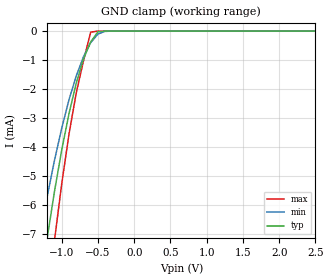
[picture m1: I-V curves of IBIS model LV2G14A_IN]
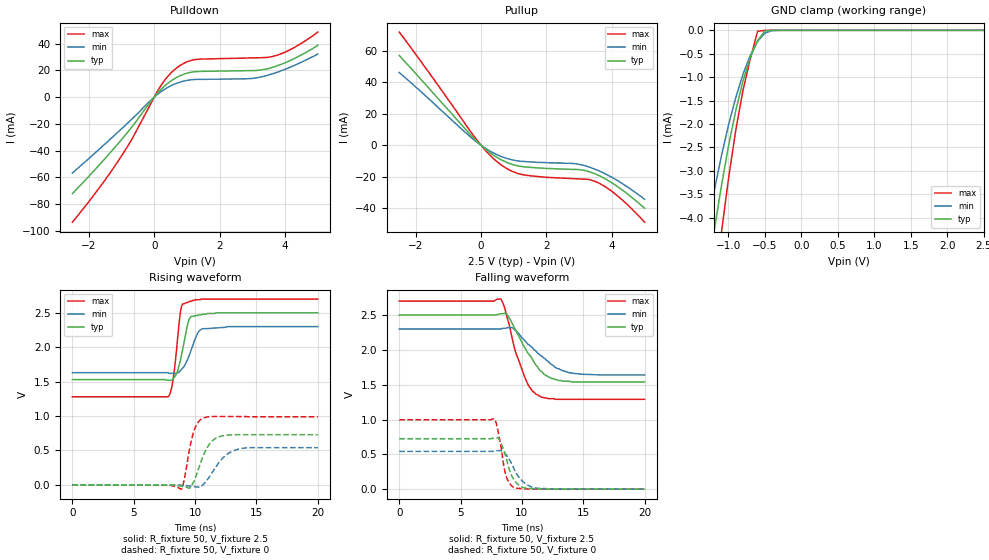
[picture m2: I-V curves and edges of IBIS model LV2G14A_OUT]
|/_/_/_/_/_/_/_/_/_/_/_/_/_/_/_/_/_/_/_/_/_/_/_/_/_/_/_/_/_/_/_/_/_/_/_/_/_/
|   Renesas Electronics Corp.
|   Multi Purpose Semiconductor Digital IC Design Group
|   IBIS Model of HD74LV2G14A
|   2.5V Triple Inverters with Schmitt-trigger Inputs,
|   SSOP-8(8pin) Package
|   History
|   V1.0   April   1, 2003   : First release.
|/_/_/_/_/_/_/_/_/_/_/_/_/_/_/_/_/_/_/_/_/_/_/_/_/_/_/_/_/_/_/_/_/_/_/_/_/_/
[IBIS Ver]   2.1
[Comment Char]  |_char
[File name]   l2g14s2.ibs
[File Rev]   1.1
[Date]   April 1, 2003
[Source]   Data created from SPICE simulations at
|   Renesas Electronics Corp.
[Notes]   RLC value of the Package is determined by assuming typical
|   conditions.
[Disclaimer]   This information is for modeling purposes only, and is not
|   guaranteed.
[Copyright]   Copyright 2003, Renesas Electronics Corp.,
|   All Rights Reserved.
|   Component  HD74LV2G14A
[Component]   HD74LV2G14A
[Manufacturer]  Renesas Electronics Corp.
[Package]
|   typ   min   max
R_pkg   0.099   0.095   0.102
L_pkg   1.740nH   1.680nH   1.790nH
C_pkg   0.140pF   0.140pF   0.150pF
[Pin]   signal_name   model_name   R_pin   L_pin   C_pin
1   1A   LV2G14A_IN   0.102   1.780nH   0.140pF
2   3Y   LV2G14A_OUT   0.097   1.710nH   0.150pF
3   2A   LV2G14A_IN   0.095   1.680nH   0.150pF
4   GND   GND   0.102   1.790nH   0.140pF
5   2Y   LV2G14A_OUT   0.101   1.790nH   0.140pF
6   3A   LV2G14A_IN   0.097   1.710nH   0.150pF
7   1Y   LV2G14A_OUT   0.097   1.710nH   0.150pF
8   VCC   POWER   0.102   1.790nH   0.140pF
| Models and submodels in the file (2): LV2G14A_IN (Input), LV2G14A_OUT (Output)
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|   Model  LV2G14A_IN
[Model]   LV2G14A_IN
Model_type  Input
Vinl = 0.75V
Vinh = 1.75V
| variable   typ   min   max
C_comp   2.85pF   2.75pF   2.95pF
| variable   typ   min   max
[Temperature range]   25   85   -40
| variable   typ   min   max
[Voltage range]   2.5V   2.3V   2.7V
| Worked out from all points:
|   GND clamp passes 1 mA (typ) near -0.70 V on its own axis
[GND Clamp]
|   Voltage   I(typ)   I(min)   I(max)
-2.5V     -38.3mA    -30.7mA    -49.7mA
-1.3V     -8.88mA    -7.07mA    -11.7mA
-1.2V     -7.13mA    -5.7mA     -9.39mA
-1.1V     -5.53mA    -4.46mA    -7.22mA
-1V       -4.1mA     -3.35mA    -5.27mA
-900mV    -2.85mA    -2.37mA    -3.56mA
-800mV    -1.8mA     -1.55mA    -2.14mA
-700mV    -962uA     -887uA     -1.03mA
-600mV    -372uA     -399uA     -36.9uA
-500mV    -22uA      -101uA     -445nA
-400mV    -433nA     -10.3uA    -2.54nA
2.5V      5.09pA     27.7pA     5pA
|   Model  LV2G14A_OUT
[Model]   LV2G14A_OUT
Model_type  Output
Polarity   Inverting
Vmeas = 1.25V
| variable   typ   min   max
C_comp   5.35pF   5.25pF   5.45pF
| variable   typ   min   max
[Temperature range]   25   85   -40
| variable   typ   min   max
[Voltage range]   2.5V   2.3V   2.7V
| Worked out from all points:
|   slope of the pulldown table from 0 to 0.375 V, typ, clamps not added: 39.2 ohm
|   slope of the pullup table from 0 to 0.375 V, typ, clamps not added: 60.8 ohm
|   GND clamp passes 1 mA (typ) near -0.78 V on its own axis
|   rising waveform, R_fixture 50, V_fixture 2.5: 20-80 % time 680ps typ, 880ps min, 506ps max; typ from 1.53 V to 2.5 V
|   rising waveform, R_fixture 50, V_fixture 0: 20-80 % time 1.02ns typ, 1.39ns min, 682ps max; typ from 0 V to 0.729 V
|   falling waveform, R_fixture 50, V_fixture 2.5: 20-80 % time 1.95ns typ, 2.56ns min, 1.45ns max; typ from 2.5 V to 1.54 V
|   falling waveform, R_fixture 50, V_fixture 0: 20-80 % time 845ps typ, 1.15ns min, 603ps max; typ from 0.724 V to 0 V
[Pullup]
|   Voltage   I(typ)   I(min)   I(max)
-2.5V     56.9mA     46.1mA     71.7mA
-200mV    4.01mA     3.18mA     5.31mA
200mV     -3.53mA    -2.75mA    -4.76mA
500mV     -7.83mA    -6.06mA    -10.6mA
900mV     -11.7mA    -8.98mA    -16mA
1.2V      -13.3mA    -10.1mA    -18.3mA
2.9V      -15.3mA    -11.7mA    -21.2mA
3.3V      -16.7mA    -13.7mA    -21.6mA
3.5V      -18.2mA    -15.3mA    -23mA
4.1V      -25.1mA    -21.5mA    -30.8mA
4.5V      -31.2mA    -26.7mA    -38.1mA
5V        -39.9mA    -34.2mA    -48.7mA
[Pulldown]
|   Voltage   I(typ)   I(min)   I(max)
-2.5V     -72mA      -56.7mA    -93.4mA
-1.7V     -51.2mA    -39.3mA    -68.5mA
-1.1V     -34.6mA    -25.9mA    -47.7mA
-700mV    -22.8mA    -16.8mA    -32.2mA
200mV     5.59mA     3.93mA     8.44mA
700mV     14.9mA     10.5mA     22.1mA
1V        17.9mA     12.5mA     26.4mA
1.3V      19.1mA     13.3mA     28.2mA
2.9V      19.8mA     13.8mA     29.3mA
3.7V      22.9mA     18.1mA     30.9mA
4.3V      29.1mA     23.9mA     37.3mA
5V        38.7mA     32.2mA     48.6mA
[GND Clamp]
|   Voltage   I(typ)   I(min)   I(max)
-2.5V     -23.4mA    -18.8mA    -30.3mA
-1.3V     -5.4mA     -4.31mA    -7.13mA
-1.2V     -4.33mA    -3.47mA    -5.69mA
-1.1V     -3.36mA    -2.71mA    -4.37mA
-1V       -2.48mA    -2.03mA    -3.18mA
-900mV    -1.72mA    -1.44mA    -2.14mA
-800mV    -1.08mA    -936uA     -1.28mA
-700mV    -575uA     -533uA     -610uA
-600mV    -219uA     -237uA     -20.5uA
-500mV    -12.9uA    -58.6uA    -245nA
-400mV    -248nA     -6.13uA    -1.4nA
2.5V      2.62pA     30.9pA     2.5pA
[Ramp]
| variable   typ   min   max
dV/dt_r   0.432/997.3p   0.325/1.398n   0.593/680.1p
dV/dt_f   0.578/1.960n   0.400/2.553n   0.847/1.445n
R_load = 50ohms
[Rising Waveform]
R_fixture = 50
V_fixture = 2.5
V_fixture_min = 2.3
V_fixture_max = 2.7
C_fixture = 0p
|   Time   V(typ)   V(min)   V(max)
0s        1.53V      1.63V      1.28V
7.8ns     1.52V      1.63V      1.28V
8.2ns     1.54V      1.62V      1.52V
8.5ns     1.62V      1.63V      1.99V
8.8ns     1.81V      1.66V      2.51V
9ns       1.98V      1.7V       2.63V
9.5ns     2.4V       1.87V      2.66V
10.2ns    2.46V      2.2V       2.69V
10.6ns    2.48V      2.27V      2.7V
20ns      2.5V       2.3V       2.7V
[Rising Waveform]
R_fixture = 50
V_fixture = 0
C_fixture = 0p
|   Time   V(typ)   V(min)   V(max)
0s        612nV      -567nV     4.06nV
8.9ns     -20.7mV    -5.82mV    -59.8mV
9.6ns     -45.5mV    -18.6mV    568mV
9.8ns     18.3mV     -23mV      723mV
10.1ns    141mV      -29.4mV    868mV
10.6ns    395mV      -3.53mV    964mV
11.6ns    667mV      237mV      994mV
12.4ns    718mV      414mV      994mV
13.4ns    729mV      513mV      993mV
20ns      729mV      540mV      989mV
[Falling Waveform]
R_fixture = 50
V_fixture = 2.5
V_fixture_min = 2.3
V_fixture_max = 2.7
C_fixture = 0p
|   Time   V(typ)   V(min)   V(max)
0s        2.5V       2.3V       2.7V
8.3ns     2.52V      2.3V       2.73V
8.8ns     2.51V      2.32V      2.46V
9.6ns     2.24V      2.26V      1.91V
10.5ns    1.95V      2.08V      1.5V
11.1ns    1.79V      1.99V      1.37V
11.8ns    1.65V      1.88V      1.31V
12.4ns    1.59V      1.79V      1.3V
13.9ns    1.55V      1.67V      1.29V
20ns      1.54V      1.64V      1.29V
[Falling Waveform]
R_fixture = 50
V_fixture = 0
C_fixture = 0p
|   Time   V(typ)   V(min)   V(max)
0s        724mV      542mV      997mV
7.7ns     733mV      545mV      1.01V
8ns       736mV      552mV      875mV
8.3ns     661mV      551mV      601mV
8.7ns     460mV      497mV      193mV
9ns       265mV      416mV      82.1mV
9.4ns     123mV      273mV      20.6mV
10.1ns    23.1mV     105mV      6.17mV
11.2ns    4.67mV     14.1mV     502uV
20ns      -2.26uV    -8.42uV    -216nV
